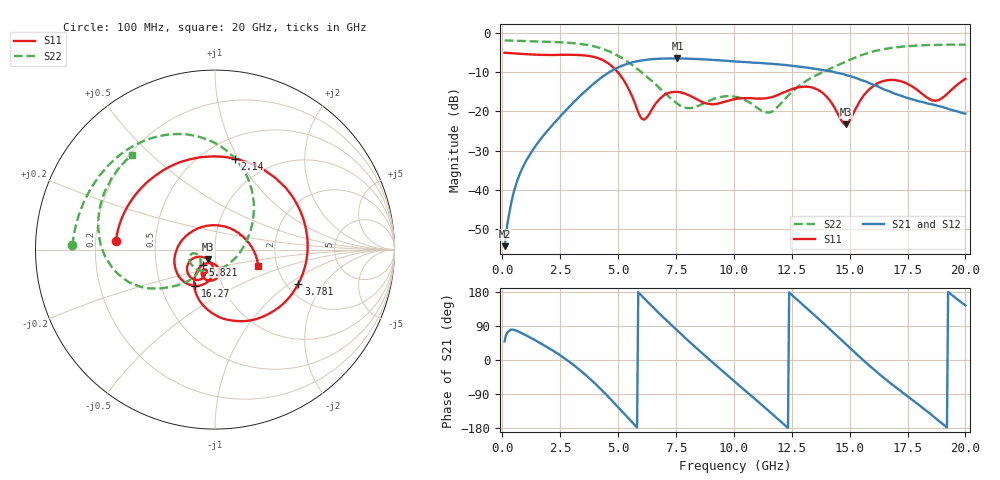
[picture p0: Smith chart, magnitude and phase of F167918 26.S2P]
!  2-Port S-parameters saved by WinCal
! VAR MeasName=S-Parameters (CALIBRATED_DATA) read from VNA (N5242A)
! VAR MeasDate=2016-11-22 10:26:00
! VAR NAME=F167918 26
! VAR FILENAME=F167918 26.S2P
! VAR DATE=2016-11-22 10:26:00
! VAR PHYS_PORTS=1,2
# Hz S DB R 50
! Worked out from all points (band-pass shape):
!   401 points, 100 MHz to 20 GHz, reference 50 ohm
!   highest |S21| = -6.58 dB at 7.562 GHz (marker M1); lowest = -54.3 dB at 100 MHz (marker M2)
!   |S21| within 3 dB of the highest: 4.766 GHz to 13.9 GHz (9.13 GHz wide, 97.8 % of centre)
!   lowest |S11| = -23.3 dB at 14.83 GHz (marker M3), VSWR 1.15, Z = 45.8 - j5.03 ohm
!   |S11| at or under -10 dB: 4.977 GHz to end of sweep
!   |S22| runs from -20.4 to -2.0 dB; largest |S21 - S12| = 0.0044
!   S11 on the Smith chart (normalised r, x): 100 MHz: 0.29, +0.04; 2.14 GHz: 0.70, +0.97; 3.781 GHz: 2.32, -1.18; 5.821 GHz: 0.87, -0.15; 16.27 GHz: 0.74, -0.32; 20 GHz: 1.60, -0.31
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1e8  -5.13 175.2  -54.31 49.0  -53.99 49.3  -2.00 178.3
7.4675e8  -5.38 145.0  -36.09 73.7  -36.06 73.6  -2.11 168.0
2.13975e9  -5.70 77.8  -23.69 26.4  -23.69 26.2  -2.37 145.4
3.43325e9  -5.75 0.8  -15.70 -30.7  -15.70 -30.6  -2.94 119.0
3.7815e9  -5.99 -22.2  -13.84 -49.3  -13.82 -49.2  -3.28 110.4
4.52775e9  -7.64 -73.5  -10.42 -93.9  -10.39 -93.9  -4.56 89.6
5.12475e9  -11.09 -110.8  -8.54 -132.6  -8.53 -132.7  -6.33 72.0
5.82125e9  -19.48 -128.3  -7.27 -178.1  -7.26 -178.3  -9.18 51.9
6.1695e9  -21.97 -95.9  -6.95 160.1  -6.95 159.9  -10.85 41.5
6.7665e9  -17.08 -81.1  -6.64 123.5  -6.65 123.5  -13.97 21.4
7.5625e9  -15.09 -105.2  -6.58 77.4  -6.58 77.4  -18.10 -20.3
8.80625e9  -18.01 -118.6  -6.84 8.5  -6.83 8.5  -17.64 -110.4
1.005e10  -16.90 -111.7  -7.32 -57.6  -7.32 -57.5  -16.31 -159.5
1.09455e10  -16.78 -116.2  -7.68 -104.5  -7.64 -104.5  -18.83 -169.2
1.189075e10  -15.86 -112.1  -8.08 -155.1  -8.05 -155.0  -18.89 -134.5
1.338325e10  -14.00 -139.3  -9.09 123.7  -9.06 123.9  -11.39 -134.5
1.4826e10  -23.32 -126.9  -10.77 42.4  -10.72 42.6  -7.37 -149.7
1.626875e10  -12.71 -118.8  -13.85 -36.6  -13.76 -36.0  -4.45 -173.6
1.67165e10  -12.07 -137.0  -14.90 -58.9  -14.88 -58.7  -3.98 178.6
1.766175e10  -13.54 177.8  -16.89 -103.4  -16.79 -103.2  -3.38 163.0
1.87065e10  -17.35 85.8  -18.46 -153.2  -18.43 -152.9  -3.14 147.7
2e10  -11.76 -20.8  -20.61 144.0  -20.46 144.5  -3.09 131.1
